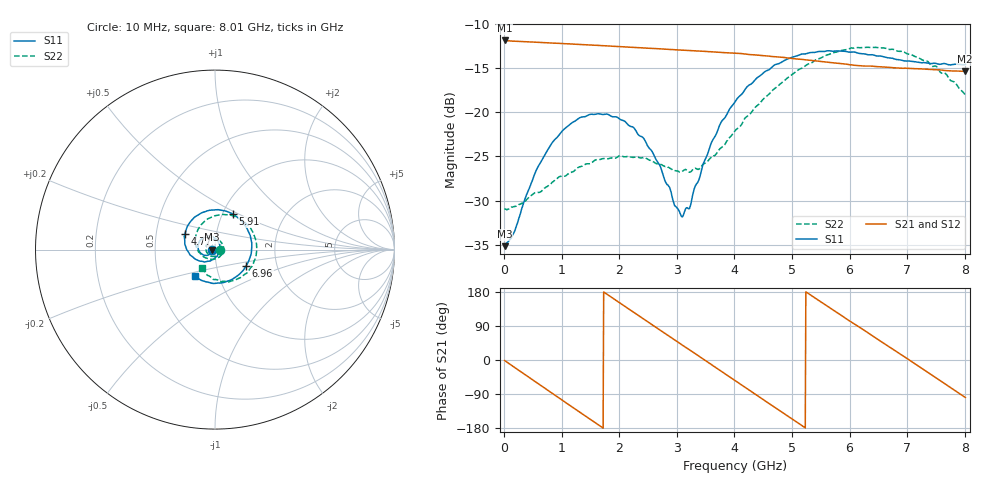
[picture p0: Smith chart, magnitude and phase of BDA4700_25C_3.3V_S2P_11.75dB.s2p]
!Agilent Technologies,E5071B,MY42404982,A.09.10
!Date: Mon Oct 20 18:07:57 2025
!Data & Calibration Information:
!Freq	S11:SOLT2(ON)	S21:SOLT2(ON)	S12:SOLT2(ON)	S22:SOLT2(ON)
# Hz S RI R 50
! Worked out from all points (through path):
!   801 points, 10 MHz to 8.01 GHz, reference 50 ohm
!   highest |S21| = -11.86 dB at 10 MHz (marker M1); lowest = -15.4 dB at 8 GHz (marker M2)
!   group delay of S21, straight-line fit = 283 ps
!   lowest |S11| = -35.2 dB at 10 MHz (marker M3), VSWR 1.04, Z = 48.3 - j0.1 ohm
!   |S11| at or under -10 dB: start of sweep to end of sweep
!   |S22| runs from -31.1 to -12.6 dB; largest |S21 - S12| = 0.003
!   S11 on the Smith chart (normalised r, x): 10 MHz: 0.97, -0.00; 4.77 GHz: 0.71, +0.13; 5.91 GHz: 1.12, +0.47; 6.96 GHz: 1.39, -0.26; 8.01 GHz: 0.76, -0.23
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1e7  -0.0174 -0.00104  0.2552 -0.00563  0.2551 -0.00585  0.0285 -0.0014
1.6e8  -0.0182 -0.00932  0.2417 -0.075  0.2417 -0.075  0.0277 -0.00911
7.1e8  -0.0476 -0.0324  0.0649 -0.2394  0.0648 -0.2395  0.000143 -0.0373
1.02e9  -0.0753 -0.0239  -0.0719 -0.2344  -0.0719 -0.2344  -0.0267 -0.0342
1.35e9  -0.0939 0.00423  -0.1889 -0.1512  -0.1889 -0.1513  -0.0487 -0.00838
1.93e9  -0.0688 0.0645  -0.2202 0.0855  -0.2203 0.0855  -0.0283 0.0471
2.41e9  -0.0116 0.0711  -0.0772 0.2181  -0.0773 0.2182  0.0235 0.0502
2.68e9  0.0153 0.0491  0.0323 0.2268  0.032 0.2265  0.0433 0.0267
3.1e9  0.0248 -0.00621  0.1753 0.141  0.1743 0.142  0.0413 -0.0212
3.23e9  0.0182 -0.0227  0.2015 0.0973  0.2016 0.097  0.032 -0.0329
3.54e9  -0.0152 -0.0568  0.2197 -0.0227  0.2197 -0.0231  -0.00316 -0.0529
4.01e9  -0.0986 -0.0584  0.1268 -0.1751  0.127 -0.1747  -0.0697 -0.0356
4.39e9  -0.1565 -0.00197  -0.0113 -0.2106  -0.0112 -0.2112  -0.1066 0.0219
4.77e9  -0.1663 0.0883  -0.138 -0.1523  -0.1371 -0.1531  -0.0987 0.1025
5.35e9  -0.067 0.2077  -0.1926 0.0387  -0.1928 0.0376  0.0149 0.1909
5.91e9  0.0991 0.1984  -0.0703 0.1742  -0.0709 0.1737  0.1695 0.1487
6.3e9  0.1811 0.111  0.051 0.1755  0.0526 0.1742  0.2289 0.0458
6.68e9  0.2032 -0.00834  0.1464 0.1041  0.1468 0.1038  0.2175 -0.0661
6.96e9  0.1731 -0.091  0.1762 0.0236  0.1759 0.0226  0.1728 -0.1328
7.48e9  0.0419 -0.1848  0.1231 -0.1235  0.1231 -0.1237  0.0341 -0.1795
8e9  -0.1111 -0.1498  -0.0236 -0.1687  -0.0234 -0.1691  -0.0709 -0.1048
8.01e9  -0.1137 -0.1482  -0.0267 -0.1683  -0.0262 -0.1685  -0.0722 -0.1024
